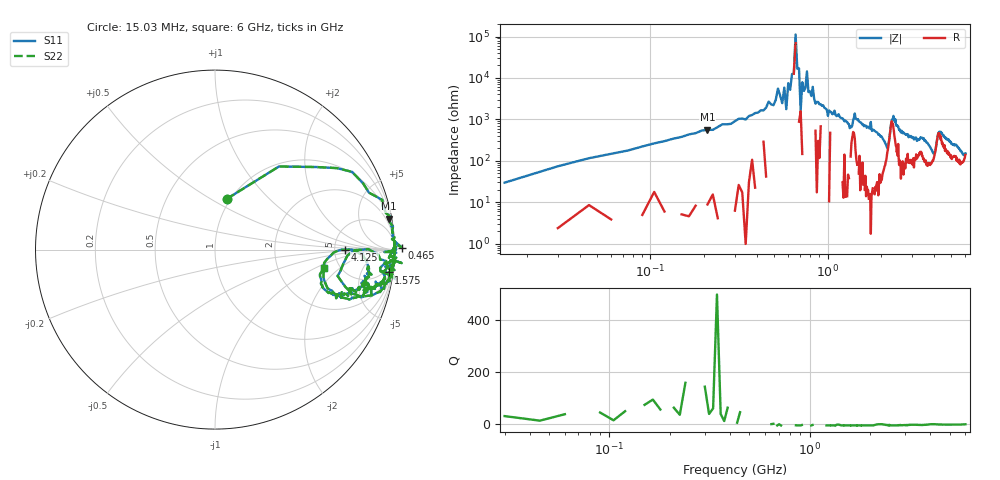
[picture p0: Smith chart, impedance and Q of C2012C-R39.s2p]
!	Network	Analyzer	HP8753E.07.74:	Oct	30	2002	Serial	No.	JP38451487
!	Hewlett-Packard
!	7	Sep	2009	12:25:46
!	Frequency	S11	S21	S12	S22
#	HZ	S	RI	R	50
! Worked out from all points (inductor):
!   400 points, 15.03 MHz to 6 GHz, reference 50 ohm
!   read as one part in series: L = 385 nH near 45.03 MHz
!   highest Q = 63.5 at 210 MHz (marker M1), where L = 425 nH
!   self-resonance near 570 MHz
!   S11 on the Smith chart (normalised r, x): 15.03 MHz: 0.96, +0.59; 465 MHz: -47, +13; 1.575 GHz: 3, -15; 4.125 GHz: 6.30, -0.04; 6 GHz: 3.77, -1.23
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1.502992e7  0.0647 0.282  0.935 -0.282  0.935 -0.282  0.0647 0.282
7.502962e7  0.764 0.433  0.236 -0.433  0.236 -0.433  0.764 0.433
2.10029e8  0.967 0.172  0.0334 -0.172  0.0334 -0.172  0.967 0.172
4.650277e8  1.04 0.0112  -0.0371 -0.0112  -0.0371 -0.0112  1.04 0.0112
5.700272e8  1 0.0171  0.000184 -0.0171  0.000184 -0.0171  1 0.0171
5.850271e8  0.969 -0.0456  0.0309 0.0456  0.0309 0.0456  0.969 -0.0456
6.00027e8  1 0.0134  -0.00048 -0.0134  -0.00048 -0.0134  1 0.0134
6.450268e8  0.992 0.00156  0.00754 -0.00156  0.00754 -0.00156  0.992 0.00156
6.600267e8  0.999 0.000701  0.00055 -0.000701  0.00055 -0.000701  0.999 0.000701
7.050265e8  0.943 -0.0135  0.0569 0.0135  0.0569 0.0135  0.943 -0.0135
7.200264e8  1 -0.0127  0.000397 0.0127  0.000397 0.0127  1 -0.0127
7.650262e8  0.996 -0.00583  0.00372 0.00583  0.00372 0.00583  0.996 -0.00583
7.800261e8  1 -0.0219  -0.00061 0.0219  -0.00061 0.0219  1 -0.0219
1.020025e9  0.996 -0.0607  0.00409 0.0607  0.00409 0.0607  0.996 -0.0607
1.575022e9  0.967 -0.127  0.0328 0.127  0.0328 0.127  0.967 -0.127
2.01002e9  0.919 -0.232  0.0815 0.232  0.0815 0.232  0.919 -0.232
2.355018e9  0.954 -0.0642  0.0456 0.0642  0.0456 0.0642  0.954 -0.0642
3.015015e9  0.892 -0.219  0.108 0.219  0.108 0.219  0.892 -0.219
4.00501e9  0.605 -0.129  0.395 0.129  0.395 0.129  0.605 -0.129
4.125009e9  0.726 -0.00134  0.274 0.00134  0.274 0.00134  0.726 -0.00134
5.010005e9  0.786 -0.225  0.214 0.225  0.214 0.225  0.786 -0.225
6e9  0.607 -0.101  0.393 0.101  0.393 0.101  0.607 -0.101
